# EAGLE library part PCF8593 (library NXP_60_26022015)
Low power clock and calendar The PCF8593 is a CMOS clock and calendar circuit, optimized for low power consumption. Addresses and data are transferred serially via the two-line bidirectional I2C-bus. The built-in word address register is incremented automatically after each written or read data byte. The built-in 32.768 kHz oscillator circuit and the first 8 bytes of the RAM are used for the clock, calendar, and counter functions. The next 8 bytes can be programmed as alarm registers or used as free RAM space. AAL Eindhoven MK
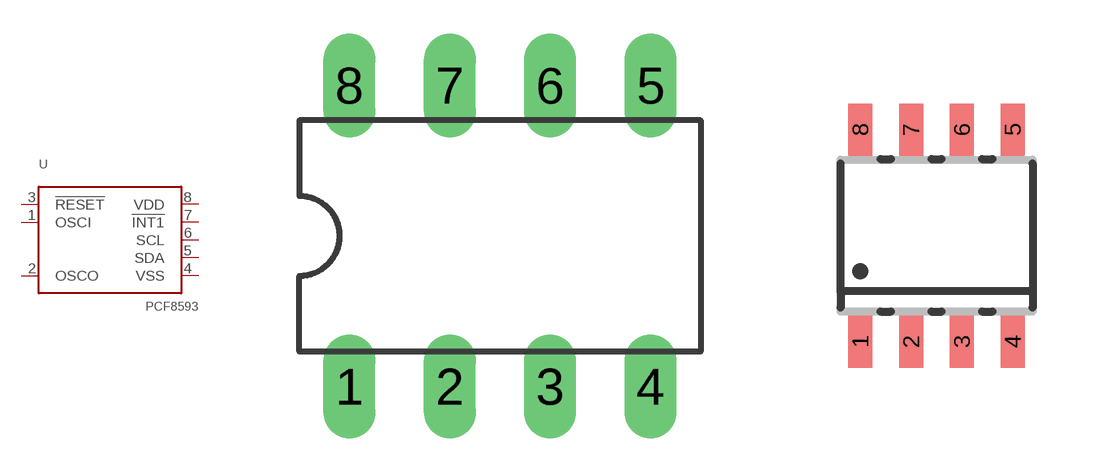
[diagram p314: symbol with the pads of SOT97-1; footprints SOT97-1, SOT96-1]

Designator prefix U

## PCF8593P  [SOT97-1]
1  OSCI  pas
2  OSCO  pas
3  !RESET  in
4  VSS  pwr
5  SDA
6  SCL  in
7  !INT1!  out
8  VDD  pwr

## PCF8593T  [SOT96-1]
Pads as for SOT97-1

## Footprint SOT97-1 (pad centres in mm)
Dual In Line Package
drill 0.813 long: 1 -3.81,-3.81; 2 -1.27,-3.81; 3 1.27,-3.81; 4 3.81,-3.81; 5 3.81,3.81; 6 1.27,3.81; 7 -1.27,3.81; 8 -3.81,3.81

## Footprint SOT96-1 (pad centres in mm)
SOT96-1 SO8: plastic small outline package; 8 leads; body width 3.9 mm JEDEC: MS-012 IEC: 076E03
smd 0.6 x 1.3: 1 -1.905,-2.65; 2 -0.635,-2.65; 3 0.635,-2.65; 4 1.905,-2.65; 5 1.905,2.65; 6 0.635,2.65; 7 -0.635,2.65; 8 -1.905,2.65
